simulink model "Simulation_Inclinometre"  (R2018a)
settings: Solver=VariableStepAuto  StartTime=0.0  StopTime=180  RelTol=1e-3
libraries: aerolibconvert2 x1, simulink x1

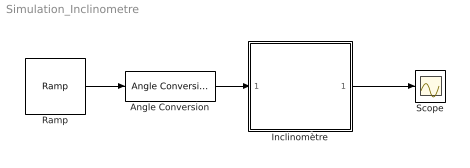
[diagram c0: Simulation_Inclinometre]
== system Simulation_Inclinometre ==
  Angle Conversion : aerolibconvert2/Angle Conversion  IU=deg  OU=rad
  Inclinomètre : Subsystem
  Ramp : simulink/Sources/Ramp  slope=1  start=0  InitialOutput=-90
  Scope : Scope
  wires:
  Inclinomètre/1(Tension) -> Scope/1
  Angle Conversion/1 -> Inclinomètre/1(Angle)
  Ramp/1 -> Angle Conversion/1

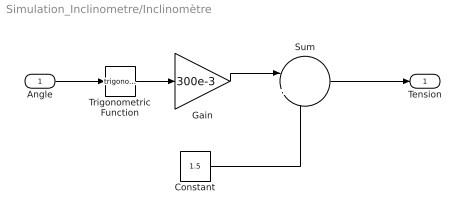
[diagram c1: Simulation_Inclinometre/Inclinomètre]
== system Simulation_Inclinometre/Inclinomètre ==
  Angle : Inport
  Constant : Constant  Value=1.5
  Gain : Gain  Gain=300e-3
  Sum : Sum  Inputs=|++
  Trigonometric Function : Trigonometry
  Tension : Outport
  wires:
  Constant/1 -> Sum/2
  Sum/1 -> Tension/1
  Gain/1 -> Sum/1
  Trigonometric Function/1 -> Gain/1
  Angle/1 -> Trigonometric Function/1
